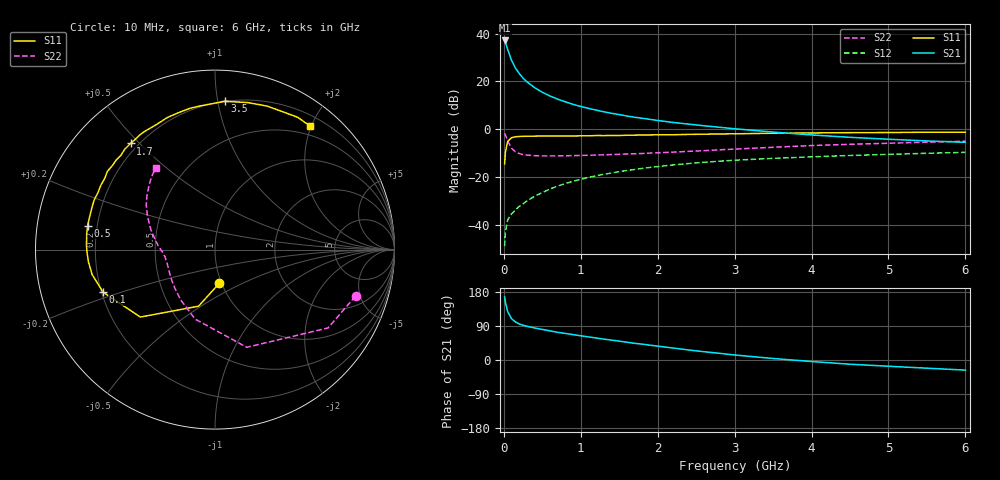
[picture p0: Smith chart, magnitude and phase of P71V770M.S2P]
! SIEMENS Small Signal Semiconductors
! BFP196
! Si NPN RF Bipolar Junction Transistor in SOT143
! VCE = 1.75 V  IC = 70 mA
! Common Emitter S-Parameters:  May  1996
# GHz  S  MA  R  50
!  f  S11  S21  S12  S22
! GHz  MAG  ANG  MAG  ANG  MAG  ANG  MAG  ANG
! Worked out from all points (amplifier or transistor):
!   36 points, 10 MHz to 6 GHz, reference 50 ohm
!   highest |S21| = 37.2 dB at 10 MHz (marker M1)
!   |S21| within 3 dB of that: start of sweep to 42.21 MHz
!   unconditionally stable (mu >= 1): 340.2 MHz to 5.215 GHz
!   at 250 MHz: K = 0.93, MSG = 26.3 dB, |S12| = -31.1 dB
!   at 1.4 GHz: K = 1.10, MAG = 10.6 dB, |S12| = -18.3 dB
!   at 6 GHz: K = 1.00, MSG = 2.1 dB, |S12| = -9.6 dB
!   S11 on the Smith chart (normalised r, x): 10 MHz: 0.98, -0.38; 100 MHz: 0.21, -0.18; 500 MHz: 0.16, +0.09; 1.7 GHz: 0.17, +0.47; 3.5 GHz: 0.20, +1.05; 6 GHz: 0.35, +1.98
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0.01  0.1888 -82.6  72.09 166.1  0.0036 78.0  0.8247 -18.3
0.02  0.3283 -106.2  66.03 152.8  0.007 67.9  0.7664 -34.7
0.05  0.5605 -137.9  46.63 127.7  0.0128 52.5  0.5724 -72.0
0.1  0.6673 -159.2  27.7 109.1  0.0171 50.9  0.4028 -105.9
0.15  0.6984 -168.5  19.25 100.6  0.0205 52.8  0.3394 -124.3
0.2  0.7084 -174.4  14.66 95.2  0.0244 56.3  0.3112 -135.7
0.25  0.7128 -178.4  11.73 91.7  0.0278 59.1  0.2964 -144.0
0.3  0.7161 178.5  9.835 89.0  0.0318 61.2  0.2888 -149.1
0.4  0.7202 173.1  7.433 84.5  0.0399 63.9  0.281 -156.9
0.5  0.7221 169.3  5.949 80.7  0.0475 65.0  0.2781 -161.8
0.6  0.7222 165.1  4.964 76.8  0.0565 65.4  0.2777 -165.1
0.7  0.7246 161.1  4.269 73.1  0.0649 65.1  0.2787 -167.6
0.9  0.7254 153.9  3.324 67.0  0.0819 63.5  0.2812 -171.7
1.1  0.7312 147.2  2.739 60.9  0.0986 61.6  0.2872 -174.5
1.4  0.7432 137.8  2.159 52.5  0.1218 57.3  0.2959 -178.2
1.7  0.7556 128.5  1.786 44.0  0.1447 53.0  0.3079 177.8
2.2  0.7689 115.3  1.392 31.6  0.1797 45.2  0.3328 171.9
2.8  0.7996 100.0  1.105 17.7  0.2153 36.0  0.3724 163.1
3.5  0.8281 86.2  0.875 4.0  0.247 25.9  0.4211 153.4
4.5  0.8506 70.1  0.68 -11.1  0.2836 13.7  0.4858 141.2
5.5  0.8693 58.0  0.571 -21.6  0.3151 2.8  0.5384 131.0
6  0.8687 52.4  0.535 -26.7  0.3298 -2.8  0.5627 126.0
